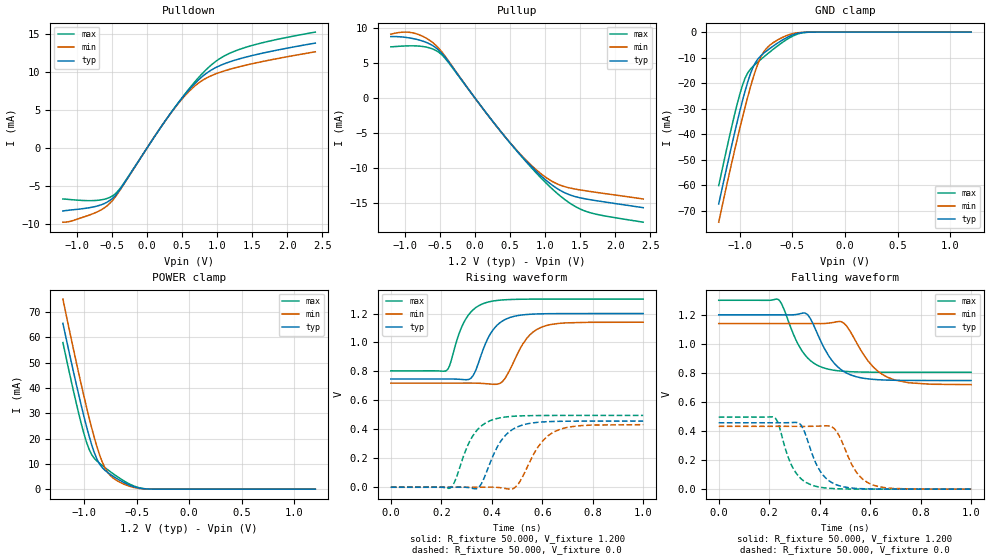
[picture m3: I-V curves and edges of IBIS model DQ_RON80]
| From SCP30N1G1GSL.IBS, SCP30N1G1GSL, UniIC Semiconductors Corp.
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|   Model DQ_RON80
[Model] DQ_RON80
Model_type I/O
Vinl =  0.500V
Vinh =  0.700V
Vmeas =  0.600V
Rref =  50.000
Vref =  0.600V
C_comp   1.373pF   1.353pF   1.403pF
[Model Spec]
Vinh   0.700V   0.670V   0.750V
Vinl   0.500V   0.470V   0.550V
Vmeas   0.600V   0.570V   0.650V
Vref   0.600V   0.570V   0.650V
Rref   50.000   NA   NA
[Temperature Range]   25.000   85.000   -40.000
[Voltage Range]   1.200V   1.140V   1.300V
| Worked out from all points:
|   slope of the pulldown table from 0 to 0.18 V, typ, clamps not added: 71.9 ohm
|   slope of the pullup table from 0 to 0.18 V, typ, clamps not added: 75.3 ohm
|   GND clamp passes 1 mA (typ) near -0.49 V on its own axis
|   POWER clamp passes 1 mA (typ) near -0.53 V on its own axis
|   rising waveform, R_fixture 50.000, V_fixture 1.200: 20-80 % time 72.8ps typ, 83.9ps min, 68.7ps max; typ from 0.748 V to 1.2 V
|   rising waveform, R_fixture 50.000, V_fixture 0.0: 20-80 % time 82.2ps typ, 90.5ps min, 76.9ps max; typ from 0 V to 0.457 V
|   falling waveform, R_fixture 50.000, V_fixture 1.200: 20-80 % time 93ps typ, 106ps min, 85.3ps max; typ from 1.2 V to 0.748 V
|   falling waveform, R_fixture 50.000, V_fixture 0.0: 20-80 % time 69.9ps typ, 77ps min, 66.2ps max; typ from 0.457 V to 0 V
[Pulldown]
|Voltage   I(typ)   I(min)   I(max)
-1.2V     -8.251mA   -9.727mA   -6.679mA
-719mV    -7.627mA   -8.41mA    -6.87mA
-571mV    -7.108mA   -7.59mA    -6.618mA
-460mV    -6.305mA   -6.506mA   -6.057mA
-349mV    -4.95mA    -5.015mA   -4.856mA
317mV     4.309mA    4.287mA    4.302mA
576mV     7.384mA    7.205mA    7.495mA
761mV     9.156mA    8.695mA    9.495mA
1.02V     10.72mA    9.858mA    11.61mA
1.279V    11.59mA    10.57mA    12.8mA
1.723V    12.59mA    11.48mA    13.97mA
2.4V      13.76mA    12.62mA    15.2mA
[Pullup]
|Voltage   I(typ)   I(min)   I(max)
-1.2V     8.762mA    9.101mA    7.299mA
-1.004V   8.671mA    9.408mA    7.423mA
-819mV    8.337mA    9.109mA    7.423mA
-634mV    7.655mA    8.151mA    7.109mA
-486mV    6.537mA    6.742mA    6.29mA
69mV      -926.2uA   -932.4uA   -913.1uA
439mV     -5.659mA   -5.646mA   -5.642mA
772mV     -9.447mA   -9.295mA   -9.571mA
1.031V    -11.88mA   -11.46mA   -12.3mA
1.29V     -13.56mA   -12.68mA   -14.55mA
1.549V    -14.34mA   -13.19mA   -16.05mA
2.4V      -15.65mA   -14.41mA   -17.72mA
[GND_clamp]
|Voltage   I(typ)   I(min)   I(max)
-1.2V     -67.26mA   -74.42mA   -60.1mA
-1.05V    -39.62mA   -46.47mA   -32.4mA
-1V       -31.05mA   -37.77mA   -24.37mA
-950mV    -23.16mA   -29.46mA   -18.1mA
-925mV    -19.62mA   -25.5mA    -16.02mA
-875mV    -13.89mA   -18.21mA   -13.48mA
-825mV    -10.4mA    -12.16mA   -11.61mA
-775mV    -8.365mA   -7.964mA   -9.852mA
-700mV    -6.001mA   -4.671mA   -7.319mA
-525mV    -1.587mA   -933.3uA   -2.208mA
-375mV    -90.13uA   -49.22uA   -132.9uA
1.2V      0A         0A         0A
[POWER_clamp]
|Voltage   I(typ)   I(min)   I(max)
-1.2V     65.51mA    75.11mA    57.91mA
-1.05V    37.38mA    45.87mA    29.99mA
-1V       28.74mA    36.73mA    21.95mA
-950mV    20.85mA    28.08mA    15.65mA
-925mV    17.34mA    24.01mA    13.56mA
-875mV    11.74mA    16.61mA    11.06mA
-825mV    8.457mA    10.65mA    9.317mA
-775mV    6.603mA    6.7mA      7.708mA
-725mV    5.177mA    4.492mA    6.178mA
-550mV    1.336mA    943.1uA    1.707mA
-400mV    85.95uA    67.55uA    91.19uA
1.2V      0A         0A         0A
[Ramp]
| variable   typ   min   max
dV/dt_r   0.274/82.196p   0.259/90.286p   0.298/77.431p
dV/dt_f   0.271/93.267p   0.252/0.106n   0.297/85.719p
R_load = 50.000
[Rising Waveform]
R_fixture= 50.000
V_fixture= 1.200
V_fixture_min= 1.140
V_fixture_max= 1.300
|time   V(typ)   V(min)   V(max)
0s        747.7mV    719.2mV    804.3mV
221ps     748mV      719.2mV    806.7mV
236ps     747.9mV    719.2mV    855.6mV
279ps     745mV      719.5mV    1.1V
319ps     756mV      719.6mV    1.214V
376ps     996.2mV    715.5mV    1.275V
442ps     1.148V     730mV      1.294V
539ps     1.193V     1.029V     1.299V
598ps     1.198V     1.107V     1.3V
1ns       1.2V       1.14V      1.3V
[Rising Waveform]
R_fixture= 50.000
V_fixture= 0.0
V_fixture_min= 0.0
V_fixture_max= 0.0
|time   V(typ)   V(min)   V(max)
0s        53.9nV     173.1nV    31.31nV
236ps     69.43uV    -7.274uV   -4.48mV
254ps     310.7uV    -23.63uV   42.05mV
307ps     -2.325mV   -14.72uV   297.5mV
349ps     214.9uV    285.9uV    407.7mV
416ps     258.5mV    -148.7uV   472.8mV
493ps     410mV      -369.9uV   491.1mV
577ps     447.6mV    262mV      495.2mV
644ps     454.5mV    380.7mV    496mV
1ns       457mV      432.4mV    496.2mV
[Falling Waveform]
R_fixture= 50.000
V_fixture= 1.200
V_fixture_min= 1.140
V_fixture_max= 1.300
|time   V(typ)   V(min)   V(max)
0s        1.2V       1.14V      1.3V
237ps     1.2V       1.14V      1.304V
313ps     1.204V     1.14V      1.002V
352ps     1.202V     1.14V      903.4mV
419ps     967.3mV    1.14V      833mV
496ps     809.4mV    1.142V     811.1mV
591ps     759.2mV    883.8mV    805.4mV
669ps     750.6mV    770mV      804.5mV
754ps     748.3mV    732mV      804.3mV
1ns       747.7mV    719.4mV    804.3mV
[Falling Waveform]
R_fixture= 50.000
V_fixture= 0.0
V_fixture_min= 0.0
V_fixture_max= 0.0
|time   V(typ)   V(min)   V(max)
0s        457mV      432.5mV    496.2mV
221ps     456.9mV    432.5mV    493.4mV
285ps     458.2mV    432.4mV    178mV
322ps     448.6mV    432.1mV    78.83mV
379ps     201.9mV    433.1mV    22.05mV
413ps     97.5mV     435.5mV    10.36mV
457ps     37.13mV    418mV      3.865mV
543ps     5.502mV    122.6mV    564.2uV
610ps     1.265mV    29.24mV    125.3uV
1ns       263.1nV    5.697uV    45.07nV
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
